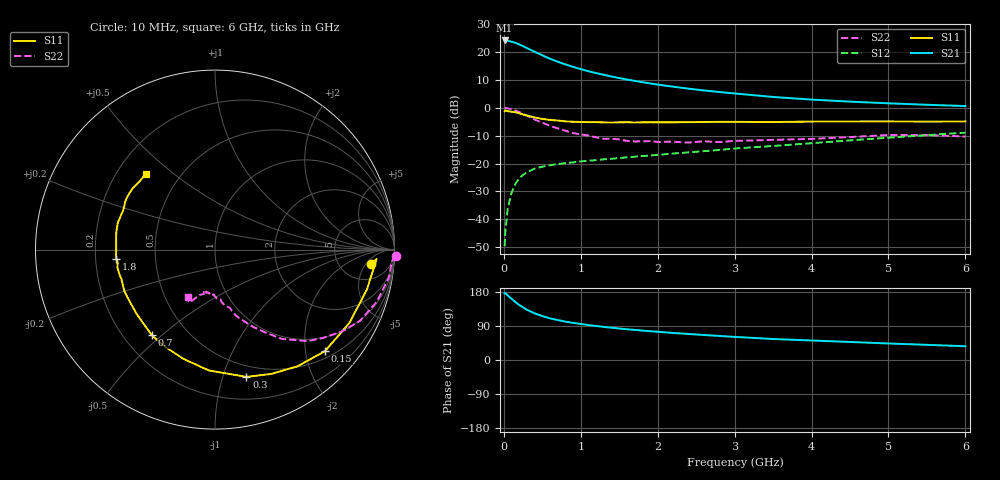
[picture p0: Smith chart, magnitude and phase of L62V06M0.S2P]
!  INFINEON TECHNOLOGIES Small Signal Semiconductors
! BFR380L3 , Si-NPN RF-Transistor in TSLP-3-1
!  Vce=2 V,  Ic=6 mA
! Common Emitter S-Parameters:  07. March 2005
#  GHz  S  MA  R  50
! f  S11  S21  S12  S22
! GHz  Mag  Ang  Mag  Ang  Mag  Ang  Mag  Ang
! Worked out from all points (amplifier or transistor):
!   36 points, 10 MHz to 6 GHz, reference 50 ohm
!   highest |S21| = 24.2 dB at 10 MHz (marker M1)
!   |S21| within 3 dB of that: start of sweep to 320.2 MHz
!   unconditionally stable (mu >= 1): 2.314 GHz to 4.773 GHz
!   at 250 MHz: K = 0.19, MSG = 23.1 dB, |S12| = -24.1 dB
!   at 1.4 GHz: K = 0.80, MSG = 14.8 dB, |S12| = -18.3 dB
!   at 6 GHz: K = 0.95, MSG = 4.8 dB, |S12| = -8.9 dB
!   S11 on the Smith chart (normalised r, x): 10 MHz: 10, -7; 150 MHz: 0.65, -2.41; 300 MHz: 0.39, -1.20; 700 MHz: 0.32, -0.47; 1.8 GHz: 0.29, -0.04; 6 GHz: 0.32, +0.40
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0.01  0.8703 -5.4  16.22 176.4  0.0033 81.7  1.01 -1.9
0.02  0.9021 -3.3  16.13 176.5  0.006 89.4  0.988 -3.7
0.05  0.8751 -14.8  16.02 170.5  0.0155 85.1  0.9816 -9.1
0.1  0.8529 -28.7  15.43 161.6  0.0301 75.8  0.9474 -17.9
0.15  0.834 -42.7  14.74 152.9  0.0432 68.7  0.8999 -26.2
0.2  0.7963 -54.7  13.78 145.2  0.0544 63.9  0.8429 -32.7
0.25  0.7605 -65.6  12.82 138.8  0.0627 58.8  0.7786 -39.2
0.3  0.7305 -76.1  11.84 132.6  0.0702 54.9  0.7263 -44.6
0.4  0.6743 -92.9  10.18 123.1  0.0812 49.0  0.6205 -53.3
0.5  0.6335 -106.2  8.768 116.0  0.0882 46.0  0.5394 -58.8
0.6  0.6082 -117.6  7.62 109.9  0.0936 43.5  0.4785 -63.9
0.7  0.593 -126.3  6.744 105.4  0.0984 42.8  0.4286 -68.1
0.9  0.5642 -141.3  5.433 97.9  0.1051 41.9  0.3528 -74.7
1.1  0.5556 -151.0  4.553 92.2  0.1125 42.7  0.3191 -79.6
1.4  0.5465 -162.5  3.651 85.3  0.1221 44.4  0.2789 -85.0
1.8  0.5511 -174.8  2.896 77.6  0.1366 47.6  0.2509 -92.3
2.2  0.551 177.0  2.403 71.4  0.1515 50.3  0.2473 -97.0
2.8  0.561 166.0  1.927 63.5  0.176 54.3  0.2437 -104.8
3.5  0.5569 156.1  1.57 55.4  0.2073 56.3  0.2671 -108.7
4.5  0.5708 148.0  1.295 47.6  0.2612 59.3  0.2993 -112.9
5.5  0.5668 138.1  1.137 40.0  0.3243 58.8  0.3258 -116.9
6  0.5711 132.3  1.079 36.3  0.3595 57.6  0.3063 -119.4
